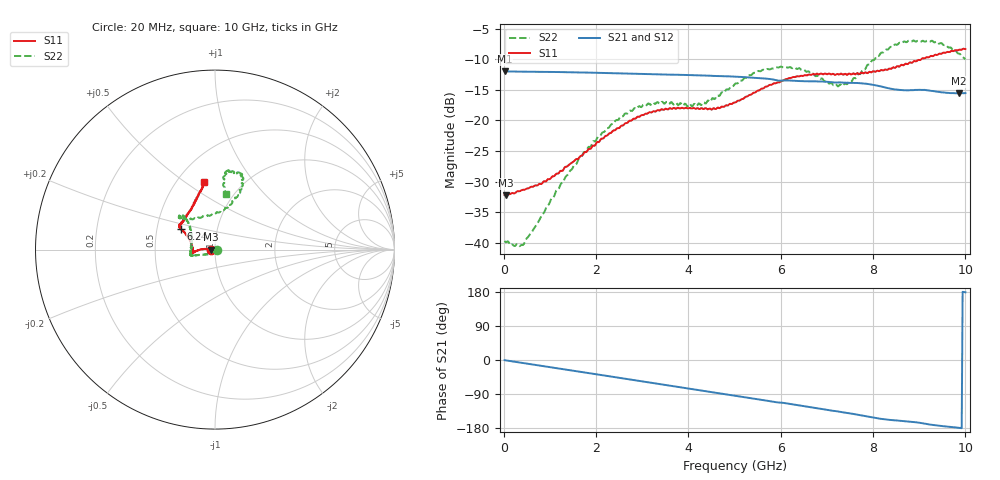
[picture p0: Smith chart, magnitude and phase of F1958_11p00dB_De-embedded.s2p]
! Integrated Device Technology
! Corporate Headquarters
! 6024 Silver Creek Valley Road
! San Jose, CA 95138  USA
! Phone:  1-408-284-8200
! Toll Free:  1-800-223-1366
! Webpage:  http://www.idt.com/
! Timing and RF Division
! 515 Groton Road, Suite 102
! Westford, MA 01886-6024
! Device:  F1958
! Description: 7-bit 0.25 dB Digital Step Attenuator
! Frequency:  0.001 -  6.000 GHz
! Package:  4x4 mm Thin QFN Plastic Package: 24 pin
! Ports:  2 RF, 12 DC
!  Pin  1  = D0
!  Pin  2  = VDD
!  Pin  3  = VMODE
!  Pin  4  = GND
!  Pin  5  = RF1  =  Port 1
!  Pin  6  = GND
!  Pin  7  = GND
!  Pin  8  = GND
!  Pin  9  = GND
!  Pin 10  = GND
!  Pin 11  = GND
!  Pin 12  = GND
!  Pin 13  = GND
!  Pin 14  = RF2  =  Port 2
!  Pin 15  = GND
!  Pin 16  = LE
!  Pin 17  = CLK
!  Pin 18  = DATA
!  Pin 19  = D6
!  Pin 20  = D5
!  Pin 21  = D4
!  Pin 22  = D3
!  Pin 23  = D2
!  Pin 24  = D1
! State:  44
! Atten State:  11.00 dB
! Voltage:  +3.30 Volts
! Current:  0.258 mA
! Data:  The device was measured on a F1958 evaluation board which has
!  individual transmission lines to the RF pins.  Data was collected
!  using a calibrated network analyzer.  The evaluation board was
!  de-embedded using Automatic Fixture Removal (AFR).
!  The reference plane is the edge of the package pin.
! Misc:
!  Action Tracker AT0419
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# GHz S dB R 50
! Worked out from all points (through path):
!   500 points, 20 MHz to 10 GHz, reference 50 ohm
!   highest |S21| = -11.97 dB at 20 MHz (marker M1); lowest = -15.6 dB at 9.86 GHz (marker M2)
!   group delay of S21, straight-line fit = 51.4 ps
!   lowest |S11| = -32.3 dB at 40 MHz (marker M3), VSWR 1.05, Z = 47.6 - j0.0662 ohm
!   |S11| at or under -10 dB: start of sweep to 9.044 GHz
!   |S22| runs from -40.6 to -6.9 dB; largest |S21 - S12| = 0.00072
!   S11 on the Smith chart (normalised r, x): 20 MHz: 0.95, -0.00; 6.24 GHz: 0.66, +0.16; 10 GHz: 0.67, +0.60
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0.02  -32.22 -178.4  -11.97 -0.5  -11.97 -0.5  -39.72 -10.5
0.04  -32.26 -178.4  -11.98 -0.9  -11.98 -0.9  -39.94 -16.5
0.42  -31.35 175.3  -12.03 -8.0  -12.03 -8.0  -40.37 -61.7
0.96  -29.60 174.6  -12.07 -18.2  -12.06 -18.1  -33.85 -113.8
1.7  -25.74 176.4  -12.16 -31.9  -12.16 -31.9  -25.79 -150.0
2.58  -20.84 -177.4  -12.32 -48.4  -12.30 -48.5  -19.35 -163.0
2.92  -19.40 -174.8  -12.38 -54.8  -12.37 -54.9  -17.72 -165.3
3.36  -18.38 -172.0  -12.48 -63.0  -12.48 -63.2  -17.18 -166.8
4.24  -18.15 -176.1  -12.62 -79.5  -12.63 -79.5  -17.25 166.0
4.64  -17.90 175.1  -12.74 -87.0  -12.75 -87.0  -15.90 148.1
5.02  -17.07 164.0  -12.84 -94.3  -12.85 -94.3  -13.96 136.6
5.56  -14.94 152.8  -13.11 -104.6  -13.12 -104.6  -11.97 133.5
6.24  -12.99 148.7  -13.49 -116.8  -13.51 -116.8  -11.45 138.2
6.68  -12.47 146.6  -13.61 -124.8  -13.62 -124.8  -12.34 134.0
7.1  -12.47 142.5  -13.75 -133.6  -13.76 -133.4  -13.87 117.2
7.36  -12.52 139.8  -13.81 -138.3  -13.82 -138.2  -14.20 95.5
7.9  -12.14 129.3  -14.05 -149.7  -14.05 -149.8  -10.87 70.7
8.34  -11.55 119.8  -14.75 -157.8  -14.75 -157.9  -8.29 66.6
8.74  -10.80 112.7  -15.08 -161.8  -15.08 -161.7  -7.14 70.1
9.26  -9.45 104.3  -15.17 -170.8  -15.17 -170.9  -6.99 79.6
9.86  -8.45 99.3  -15.58 -178.9  -15.62 -178.9  -9.08 81.1
10  -8.32 99.3  -15.54 178.7  -15.56 178.9  -10.02 78.6
